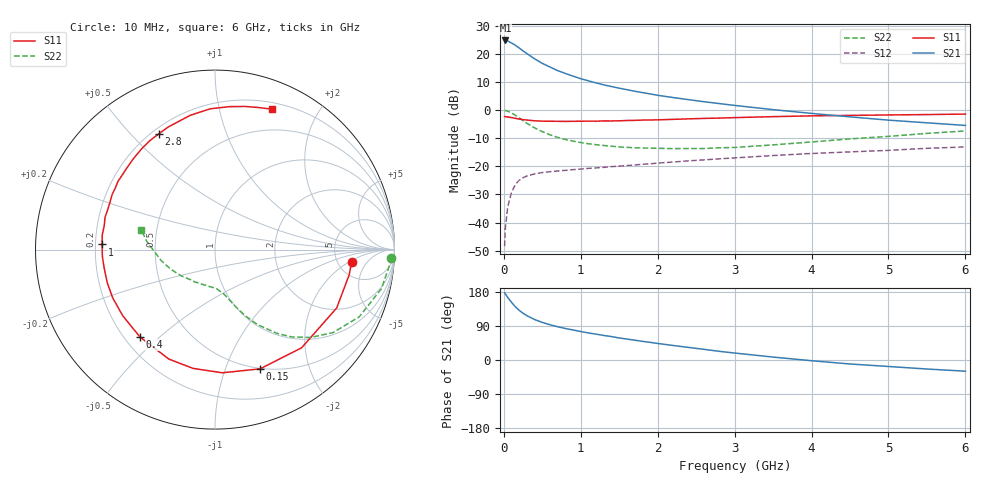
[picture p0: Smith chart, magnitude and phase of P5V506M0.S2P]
! SIEMENS Small Signal Semiconductors
! BFP183
! Si NPN RF Bipolar Junction Transistor in SOT143
! VCE = 0.5 V  IC = 6 mA
! Common Emitter S-Parameters:  March  1996
# GHz  S  MA  R  50
!  f  S11  S21  S12  S22
! GHz  MAG  ANG  MAG  ANG  MAG  ANG  MAG  ANG
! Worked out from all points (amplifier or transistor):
!   36 points, 10 MHz to 6 GHz, reference 50 ohm
!   highest |S21| = 24.7 dB at 20 MHz (marker M1)
!   |S21| within 3 dB of that: start of sweep to 215.2 MHz
!   unconditionally stable (mu >= 1): 1.216 GHz to end of sweep
!   at 250 MHz: K = 0.26, MSG = 22.5 dB, |S12| = -24.1 dB
!   at 1.4 GHz: K = 1.08, MAG = 12.5 dB, |S12| = -20.1 dB
!   at 6 GHz: K = 1.15, MAG = 1.5 dB, |S12| = -13.1 dB
!   S11 on the Smith chart (normalised r, x): 10 MHz: 6.78, -2.17; 150 MHz: 0.49, -1.33; 400 MHz: 0.26, -0.43; 1 GHz: 0.23, +0.02; 2.8 GHz: 0.23, +0.60; 6 GHz: 0.27, +1.45
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0.01  0.7644 -5.0  17.09 177.3  0.0038 84.5  0.9795 -2.6
0.02  0.761 -10.5  17.17 174.6  0.0081 79.9  0.9753 -5.4
0.05  0.752 -25.6  16.81 165.3  0.0188 77.5  0.9525 -13.2
0.1  0.7295 -48.6  15.48 152.2  0.0346 65.7  0.8866 -25.0
0.15  0.7102 -69.3  14.12 140.3  0.0475 56.5  0.804 -35.1
0.2  0.6876 -86.6  12.61 131.0  0.0564 50.3  0.7221 -42.7
0.25  0.6731 -100.5  11.17 123.3  0.0625 43.9  0.6464 -48.8
0.3  0.6619 -112.9  10.04 117.0  0.0671 40.1  0.5789 -53.6
0.4  0.6417 -130.7  8.114 106.7  0.0732 34.4  0.48 -60.5
0.5  0.6324 -144.4  6.723 99.2  0.0773 31.0  0.4124 -64.9
0.6  0.6303 -154.8  5.791 93.0  0.08 29.0  0.3624 -68.3
0.7  0.628 -163.1  4.999 87.8  0.0823 28.0  0.3248 -71.1
0.8  0.626 -170.8  4.448 83.1  0.0846 27.3  0.299 -73.3
1  0.6301 177.4  3.592 75.1  0.0889 26.5  0.2636 -77.2
1.1  0.6334 172.5  3.289 71.3  0.0916 26.7  0.2508 -79.0
1.5  0.6418 155.8  2.437 58.1  0.1004 27.2  0.2202 -87.0
2.2  0.6806 132.0  1.662 38.3  0.1188 26.8  0.2055 -104.5
2.8  0.7172 115.9  1.299 22.9  0.1354 25.0  0.2126 -121.7
3.5  0.7607 100.5  1.013 7.7  0.155 21.9  0.2396 -142.7
4.5  0.8006 84.2  0.754 -10.5  0.1799 15.5  0.3059 -168.4
5.5  0.8281 72.9  0.591 -23.8  0.2083 9.6  0.3833 173.1
6  0.8444 67.8  0.531 -29.5  0.2202 5.6  0.4239 165.2
